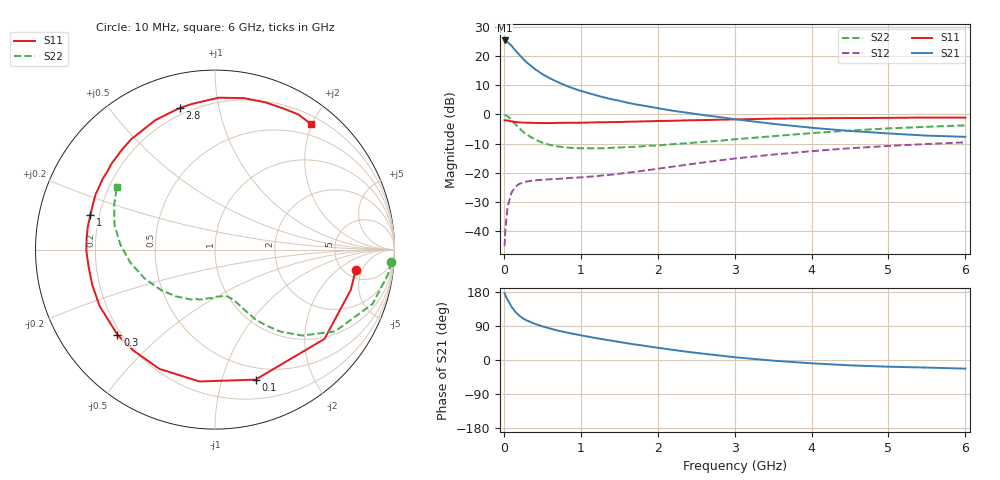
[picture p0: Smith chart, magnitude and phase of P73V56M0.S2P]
! SIEMENS Small Signal Semiconductors
! BFP196
! Si NPN RF Bipolar Junction Transistor in SOT143
! VCE = 3.5 V  IC = 6 mA
! Common Emitter S-Parameters:  May  1996
# GHz  S  MA  R  50
!  f  S11  S21  S12  S22
! GHz  MAG  ANG  MAG  ANG  MAG  ANG  MAG  ANG
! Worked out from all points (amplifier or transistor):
!   36 points, 10 MHz to 6 GHz, reference 50 ohm
!   highest |S21| = 25.4 dB at 10 MHz (marker M1)
!   |S21| within 3 dB of that: start of sweep to 136.6 MHz
!   unconditionally stable (mu >= 1): 1.042 GHz to 3.189 GHz
!   at 250 MHz: K = 0.29, MSG = 21.2 dB, |S12| = -23.4 dB
!   at 1.4 GHz: K = 1.15, MAG = 10.6 dB, |S12| = -20.7 dB
!   at 6 GHz: K = 0.99, MSG = 0.9 dB, |S12| = -9.6 dB
!   S11 on the Smith chart (normalised r, x): 10 MHz: 6.18, -3.84; 100 MHz: 0.38, -1.29; 300 MHz: 0.18, -0.36; 1 GHz: 0.17, +0.13; 2.8 GHz: 0.17, +0.77; 6 GHz: 0.32, +1.99
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0.01  0.7919 -8.4  18.57 176.5  0.0055 87.6  0.9849 -4.1
0.02  0.7889 -16.6  18.13 170.8  0.0109 80.6  0.975 -7.9
0.05  0.7872 -39.2  17.3 158.5  0.0264 70.6  0.9289 -19.0
0.1  0.7589 -72.7  15.11 140.7  0.0457 55.8  0.8091 -34.3
0.15  0.7398 -96.7  12.5 126.9  0.0575 44.9  0.6819 -44.6
0.2  0.7333 -115.0  10.61 117.3  0.0643 38.4  0.5834 -51.5
0.25  0.7232 -129.0  8.97 109.6  0.0678 33.3  0.5038 -56.4
0.3  0.7213 -138.9  7.758 104.1  0.071 30.4  0.4495 -59.9
0.4  0.7157 -153.8  6.06 95.7  0.074 26.7  0.3741 -63.9
0.5  0.7118 -163.9  4.914 88.8  0.0757 25.4  0.3281 -67.0
0.6  0.7108 -172.2  4.151 83.1  0.0773 25.2  0.2995 -69.8
0.8  0.7182 174.9  3.148 73.4  0.0803 25.8  0.2714 -74.8
1  0.7206 164.3  2.536 65.2  0.0831 28.1  0.263 -79.6
1.1  0.7258 159.7  2.317 61.4  0.0853 29.3  0.2628 -82.7
1.3  0.7344 151.4  1.965 54.3  0.0903 32.3  0.2629 -88.6
1.6  0.749 140.5  1.596 44.3  0.0997 36.2  0.2742 -97.8
2.2  0.778 121.1  1.155 26.7  0.1273 40.2  0.3096 -116.2
2.8  0.8129 104.0  0.903 12.0  0.1625 39.0  0.3536 -136.3
3.5  0.8465 88.6  0.69 -1.7  0.2048 33.3  0.4237 -157.6
4.5  0.8668 71.1  0.521 -14.1  0.2631 22.3  0.5287 176.8
5.5  0.8847 58.2  0.433 -20.0  0.3113 10.0  0.6141 156.3
6  0.8805 52.5  0.413 -22.8  0.3321 3.4  0.6485 147.3
